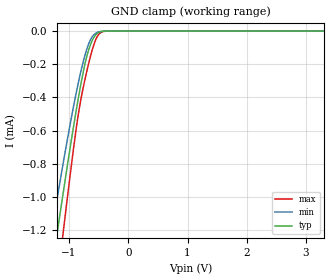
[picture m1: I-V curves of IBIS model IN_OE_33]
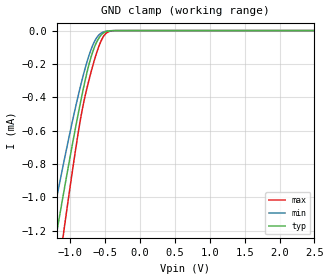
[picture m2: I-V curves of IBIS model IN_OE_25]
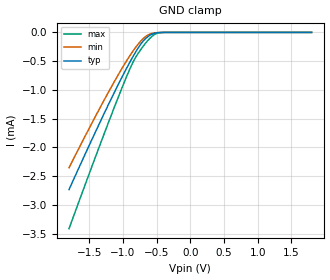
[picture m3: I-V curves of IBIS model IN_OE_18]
| TEXAS INSTRUMENTS INCORPORATED
| Standard Linear and Logic Group / High Volume Linear
| IBIS Model of TXB0302
| 2bit Auto-sensing Bi-directional level translator
| This file contains package information for the following:
|  dqm 8-pin (PW) package as [Component] TXB0302_PW
| This device can be powered at the following Vccs:
|  3.3 volt Vcc
|  2.5 volt Vcc
|  1.8 volt Vcc
|  1.5 volt Vcc
|  1.2 volt Vcc
| This file provides unique models under the [Model Selector] for each Vcc.
| For operation at a specific Vcc, select the appropriate model after each
| [Model Selector] keyword.
[IBIS Ver]   4.0
[Comment char]  |_char
[File Name]   txb0302.ibs
[File Rev]   1.1 | TXB0302A0
[Date]   June 21, 2012
[Source]   Data created from TI-SPICE simulations at TI-SLL/HVL.
   The following is an IBIS list for the TXB0302.
   Please contact sllibis@ti.com with questions and
   comments concerning SLL IBIS models.
[Notes]   Revision_History:
   - 1.1 06/21/12   Added models for one-shot circuit on
   for IO_A model
   IBIS model ver1.0 of TXB0302
   IO_A_33 pullup is non-monotonic
   IO_A_18 powerclamp and pullup is non-monotonic
   IO_A_15 pullup is non-monotonic
   IO_A_12 pullup and pulldown is non-monotonic
   Please note that models for one shot circuit on can be chosen under
   [Model Selector] for IO_A model.
[Disclaimer]
| This model is designed as an aid for customers of Texas Instruments.
| TI and its licensors and suppliers make no warranties, either expressed
| or implied, with respect to this  model, including the warranties of
| merchantability or fitness for a particular purpose. The model is
| provided solely on an "as is" basis. The entire risk as to its quality
| and performance is with the customer.
[Copyright]
| (C) Copyright 2012 Texas Instruments Incorporated. All rights reserved.
| Component TXB0302_PW 8-PIN DQM
[Component]   TXB0302_PW
[Manufacturer]   Texas Instruments, Inc.
[Package]
|   typ   min   max
R_pkg   5.165e-02   4.655e-02   5.882e-02
L_pkg   4.185e-10   3.631e-10   4.910e-10
C_pkg   5.793e-14   5.510e-14   6.206e-14
[Pin]   signal_name   model_name   R_pin   L_pin   C_pin
1   VCC   POWER   5.882e-02   4.910e-10   6.206e-14
2   A1   IO_A   4.725e-02   3.702e-10   5.574e-14
3   A2   IO_A   4.655e-02   3.631e-10   5.510e-14
4   GND   GND   5.452e-02   4.459e-10   5.898e-14
5   OE   IN_OE   5.452e-02   4.498e-10   5.904e-14
6   B2   IO_A   4.660e-02   3.697e-10   5.527e-14
7   B1   IO_A   4.703e-02   3.740e-10   5.573e-14
8   VCC   POWER   5.788e-02   4.847e-10   6.149e-14
| Model IN_OE
[Model Selector]   IN_OE
IN_OE_33   3.3 volt Vcc
IN_OE_25   2.5 volt Vcc
IN_OE_18   1.8 volt Vcc
IN_OE_15   1.5 volt Vcc
IN_OE_12   1.2 volt Vcc
| Model IO_A
[Model Selector]   IO_A
IO_A_33   3.3 volt Vcc
IO_A_25   2.5 volt Vcc
IO_A_18   1.8 volt Vcc
IO_A_15   1.5 volt Vcc
IO_A_12   1.2 volt Vcc
IO_A_OS_33   one shot circuit on at   3.3 volt Vcc
IO_A_OS_25   one shot circuit on at   2.5 volt Vcc
IO_A_OS_18   one shot circuit on at   1.8 volt Vcc
IO_A_OS_15   one shot circuit on at   1.5 volt Vcc
IO_A_OS_12   one shot circuit on at   1.2 volt Vcc
| Models and submodels in the file (15): IN_OE_33 (Input), IN_OE_25 (Input), IN_OE_18 (Input), IN_OE_15 (Input), IN_OE_12 (Input), IO_A_33 (3-state), IO_A_25 (3-state), IO_A_18 (3-state), IO_A_15 (3-state), IO_A_12 (3-state), IO_A_OS_33 (3-state), IO_A_OS_25 (3-state), IO_A_OS_18 (3-state), IO_A_OS_15 (3-state), IO_A_OS_12 (3-state)
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[Model]   IN_OE_33
Model_type  Input
Vinl=1.15
Vinh=2.15
| variable   typ   min   max
C_comp   0.32pF   0.23pF   0.40pF
[Temperature Range]   40   100   -40
| Ambient temperature   25   85   -40
[Voltage range]   3.3   3   3.6
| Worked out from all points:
|   GND clamp passes 1 mA (typ) near -1.11 V on its own axis
[GND Clamp]
| IN_OE_33
|   Voltage   I(typ)   I(min)   I(max)
-3.3V     -6.752mA   -6.005mA   -8.357mA
-1.315V   -1.499mA   -1.255mA   -1.875mA
-1.27V    -1.388mA   -1.157mA   -1.736mA
-1.195V   -1.205mA   -996.7uA   -1.505mA
-1.105V   -989.6uA   -808.7uA   -1.232mA
-1.075V   -918.9uA   -747.4uA   -1.142mA
-920mV    -566.5uA   -446.4uA   -696.5uA
-815mV    -348uA     -265.7uA   -440.9uA
-675mV    -120.7uA   -82.99uA   -203.7uA
-530mV    -15.65uA   -9.097uA   -37.64uA
-345mV    -145.2nA   -101nA     -185.5nA
3.3V      331.8pA    845pA      15.41pA
[Model]   IN_OE_25
Model_type  Input
Vinl=0.875
Vinh=1.625
| variable   typ   min   max
C_comp   0.33pF   0.23pF   0.41pF
[Temperature Range]   40   100   -40
| Ambient temperature   25   85   -40
[Voltage range]   2.5   2.3   2.7
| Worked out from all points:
|   GND clamp passes 1 mA (typ) near -1.11 V on its own axis
[GND Clamp]
| IN_OE_25
|   Voltage   I(typ)   I(min)   I(max)
-2.5V     -4.582mA   -4.021mA   -5.695mA
-1.3V     -1.462mA   -1.222mA   -1.828mA
-1.265V   -1.376mA   -1.146mA   -1.72mA
-1.195V   -1.205mA   -996.7uA   -1.505mA
-1.095V   -965.9uA   -788.1uA   -1.202mA
-920mV    -566.5uA   -446.4uA   -696.5uA
-825mV    -367.7uA   -281.7uA   -461.6uA
-690mV    -139.2uA   -97.9uA    -226.3uA
-550mV    -22.8uA    -13.11uA   -52.83uA
-480mV    -5.357uA   -3.256uA   -13.08uA
-370mV    -301.4nA   -199.5nA   -468.8nA
2.5V      194.3pA    534.3pA    11.53pA
[Model]   IN_OE_18
Model_type  Input
Vinl=0.63
Vinh=1.17
| variable   typ   min   max
C_comp   0.34pF   0.25pF   0.43pF
[Temperature Range]   40   100   -40
| Ambient temperature   25   85   -40
[Voltage range]   1.8   1.65   1.95
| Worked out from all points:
|   GND clamp passes 1 mA (typ) near -1.11 V on its own axis
[GND Clamp]
| IN_OE_18
|   Voltage   I(typ)   I(min)   I(max)
-1.8V     -2.731mA   -2.352mA   -3.411mA
-1.52V    -2.013mA   -1.71mA    -2.518mA
-1.275V   -1.4mA     -1.168mA   -1.751mA
-1.06V    -883.8uA   -717uA     -1.098mA
-915mV    -555.6uA   -437.2uA   -682.9uA
-825mV    -367.7uA   -281.7uA   -461.6uA
-720mV    -181.1uA   -131.6uA   -273.2uA
-645mV    -88.33uA   -57.42uA   -160.8uA
-565mV    -29.57uA   -17.01uA   -66.21uA
-485mV    -6.009uA   -3.638uA   -14.74uA
-385mV    -461.8nA   -298.9nA   -795.8nA
1.8V      66.55pA    352.3pA    8.466pA
